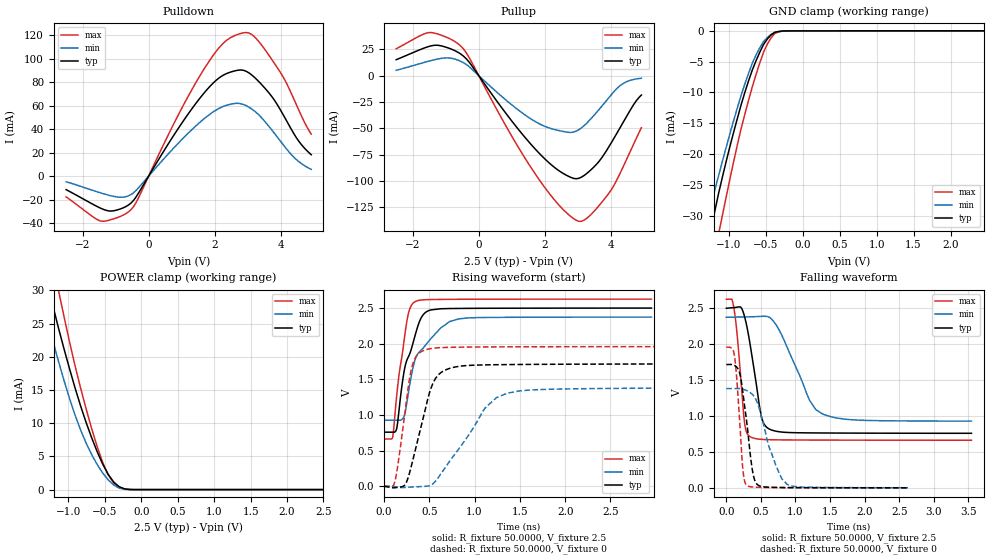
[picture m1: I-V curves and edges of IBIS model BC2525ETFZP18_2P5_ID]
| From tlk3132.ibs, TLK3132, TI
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|   Model Cell BC2525ETFZP18_2P5_ID
|BC2525ETFZP18_2P5
[Model]   BC2525ETFZP18_2P5_ID
Model_type   I/O
Polarity   Non-Inverting
Enable   Active-Low
Vinl =  0.7V
Vinh =  1.7V
Cref =  15.0000pF
Rref =  100.0000M
Vref =  0V
Vmeas =  1.25
C_comp   2.309127p   2.211398p   2.342242p
[Model Spec]
Vinl   0.7V   0.7V   0.7V
Vinh   1.7V   1.7V   1.7V
[Temperature Range]   25   125   -40
[Voltage Range]   2.5   2.375   2.625
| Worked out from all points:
|   slope of the pulldown table from 0 to 0.375 V, typ, clamps not added: 21.4 ohm
|   slope of the pullup table from 0 to 0.375 V, typ, clamps not added: 22.5 ohm
|   GND clamp passes 1 mA (typ) near -0.45 V on its own axis
|   POWER clamp passes 1 mA (typ) near -0.36 V on its own axis
|   rising waveform, R_fixture 50.0000, V_fixture 2.5: 20-80 % time 182ps typ, 269ps min, 118ps max; typ from 0.759 V to 2.5 V
|   rising waveform, R_fixture 50.0000, V_fixture 0: 20-80 % time 205ps typ, 437ps min, 126ps max; typ from 0 V to 1.72 V
|   falling waveform, R_fixture 50.0000, V_fixture 2.5: 20-80 % time 169ps typ, 384ps min, 102ps max; typ from 2.5 V to 0.76 V
|   falling waveform, R_fixture 50.0000, V_fixture 0: 20-80 % time 129ps typ, 255ps min, 80.8ps max; typ from 1.72 V to 0.001 V
[POWER_clamp]
|   voltage   I(typ)   I(min)   I(max)
-2.5V     103mA      76.93mA    125mA
-1.389V   36.5mA     29.59mA    43.69mA
-1.364V   35.11mA    28.53mA    42.23mA
-1.237V   28.84mA    23.35mA    35.36mA
-1.111V   23.3mA     18.37mA    28.69mA
-984.8mV  18.21mA    13.74mA    22.27mA
-833.3mV  12.63mA    8.998mA    15.33mA
-606.1mV  5.731mA    3.804mA    6.499mA
-454.5mV  2.303mA    1.471mA    2.232mA
-303mV    430uA      225uA      328.3uA
-75.76mV  1.022uA    1.107uA    345.1nA
2.5V      48.25nA    205.1nA    50.68nA
[Pulldown]
|   voltage   I(typ)   I(min)   I(max)
-2.5V     -11.51mA   -4.832mA   -17.68mA
-1.439V   -27.53mA   -14.42mA   -38.36mA
-1.061V   -29.57mA   -17.27mA   -36.41mA
-530.3mV  -22.86mA   -15.68mA   -28.47mA
909.1mV   41.11mA    28.35mA    52.71mA
1.667V    70.38mA    48.57mA    90.72mA
2.273V    86.19mA    59.51mA    113.6mA
2.803V    90.44mA    61.62mA    121.7mA
3.182V    84.74mA    56mA       119.3mA
3.636V    71.14mA    42.56mA    103.2mA
4.394V    36.35mA    16.16mA    65.9mA
4.924V    18.23mA    5.798mA    35.78mA
[Pullup]
|   voltage   I(typ)   I(min)   I(max)
-2.5V     15.14mA    5.153mA    25.5mA
-1.515V   27.67mA    13.72mA    40.84mA
-1.136V   28.26mA    16.39mA    38.38mA
-530.3mV  20.16mA    13.36mA    27.64mA
1.667V    -68.19mA   -42.76mA   -91.26mA
2.424V    -90.17mA   -52.1mA    -122.7mA
3.03V     -97.45mA   -51.32mA   -138.3mA
3.258V    -93.2mA    -45.49mA   -135.8mA
3.561V    -84.34mA   -35.15mA   -126.3mA
4.015V    -63.64mA   -18.09mA   -108.3mA
4.394V    -43.2mA    -7.12mA    -85.11mA
4.924V    -18.43mA   -2.488mA   -49.38mA
[GND_clamp]
|   voltage   I(typ)   I(min)   I(max)
-2.5V     -116.2mA   -88.1mA    -139.9mA
-1.338V   -38.29mA   -32.77mA   -45.06mA
-1.288V   -35.07mA   -30.4mA    -41.9mA
-1.237V   -32.01mA   -28.04mA   -38.85mA
-1.136V   -26.24mA   -23.38mA   -32.83mA
-1.086V   -23.65mA   -21.11mA   -29.86mA
-833.3mV  -11.97mA   -10.44mA   -15.84mA
-681.8mV  -6.338mA   -5.249mA   -9.062mA
-530.3mV  -2.211mA   -1.736mA   -3.463mA
-378.8mV  -238.8uA   -246.4uA   -429.3uA
-227.3mV  -10.88uA   -15.73uA   -14.61uA
2.449V    3.343nA    1.705uA    32.31nA
[Ramp]
| variable   typ   min   max
dV/dt_f   1.057973/0.1692899n  0.8798866/0.3880072n   1.18762/0.1030907n
dV/dt_r   1.045282/0.2067669n  0.8447445/0.4452987n   1.19162/0.1277788n
R_load = 50
[Rising Waveform]
R_fixture = 50.0000
V_fixture = 2.5
V_fixture_min = 2.375
V_fixture_max = 2.625
|   time   V(typ)   V(min)   V(max)
0s        759mV      927.1mV    662.8mV
96ps      758.5mV    927.1mV    688.3mV
138ps     796.3mV    927.1mV    1.237V
216ps     1.562V     964.6mV    1.983V
258ps     1.785V     1.216V     2.351V
348ps     2.135V     1.793V     2.592V
468ps     2.447V     1.994V     2.617V
624ps     2.49V      2.217V     2.621V
828ps     2.494V     2.348V     2.623V
2.952ns   2.499V     2.373V     2.625V
[Rising Waveform]
R_fixture = 50.0000
V_fixture = 0
V_fixture_min = 0
V_fixture_max = 0
|   time   V(typ)   V(min)   V(max)
0s        45.2uV     21.86uV    69.1uV
120ps     -20.23mV   -6.336mV   63.61mV
240ps     36.1mV     -15.95mV   1.115V
318ps     363.6mV    -9.228mV   1.715V
444ps     1.014V     -1.531mV   1.907V
540ps     1.444V     33.5mV     1.935V
660ps     1.619V     232.7mV    1.947V
1.116ns   1.702V     1.098V     1.954V
1.362ns   1.707V     1.305V     1.956V
4.098ns   1.716V     1.379V     1.959V
[Falling Waveform]
R_fixture = 50.0000
V_fixture = 2.5
V_fixture_min = 2.375
V_fixture_max = 2.625
|   time   V(typ)   V(min)   V(max)
0s        2.5V       2.375V     2.625V
108ps     2.509V     2.376V     2.51V
162ps     2.516V     2.378V     2.072V
264ps     2.383V     2.379V     900.4mV
348ps     1.972V     2.381V     709.6mV
510ps     971.5mV    2.388V     674.9mV
654ps     805.4mV    2.35V      669.6mV
1.2ns     765.3mV    1.225V     665.8mV
1.398ns   763.9mV    1.026V     665.2mV
3.546ns   759.6mV    929.5mV    663.2mV
[Falling Waveform]
R_fixture = 50.0000
V_fixture = 0
V_fixture_min = 0
V_fixture_max = 0
|   time   V(typ)   V(min)   V(max)
0s        1.716V     1.381V     1.96V
120ps     1.703V     1.381V     1.827V
192ps     1.601V     1.381V     944mV
240ps     1.322V     1.373V     249.2mV
300ps     876.7mV    1.352V     31.45mV
372ps     273.5mV    1.305V     12.95mV
426ps     74.17mV    1.234V     9.309mV
708ps     7.125mV    334.9mV    2.974mV
882ps     4.689mV    46.81mV    1.988mV
2.628ns   1.101mV    2.407mV    238.3uV
